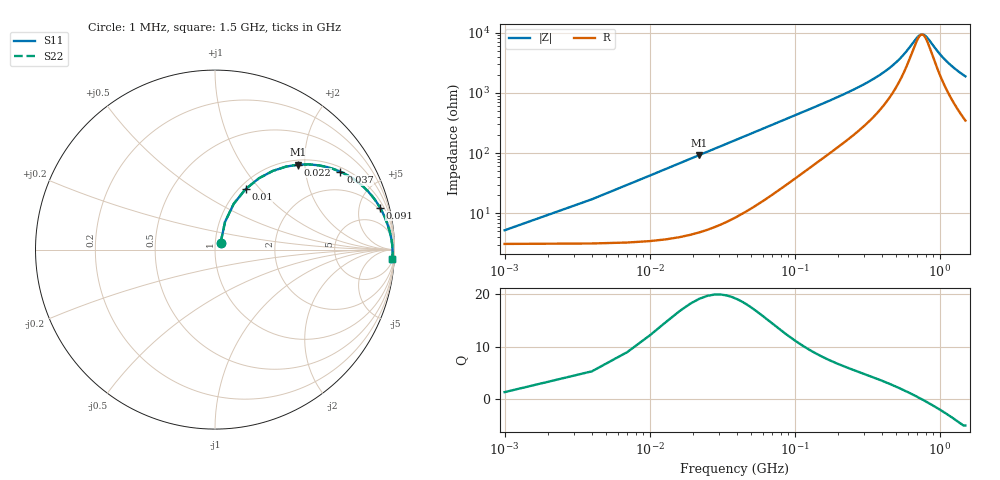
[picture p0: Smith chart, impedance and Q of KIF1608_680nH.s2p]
# MHz S RI R 50
!Freq ReS11 ImS11 ReS21 ImS21 ReS12 ImS12 ReS22 ImS22
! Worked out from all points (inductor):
!   501 points, 1 MHz to 1.5 GHz, reference 50 ohm
!   read as one part in series: L = 669 nH near 7 MHz
!   highest Q = 19.2 at 22 MHz (marker M1), where L = 669 nH
!   self-resonance near 750.9 MHz
!   S11 on the Smith chart (normalised r, x): 1 MHz: 1.06, +0.08; 10 MHz: 1.07, +0.84; 22 MHz: 1.10, +1.85; 37 MHz: 1.16, +3.11; 91 MHz: 1.64, +7.64; 1.5 GHz: 8, -37
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1  0.0317 0.0395  0.9683 -0.0395  0.9683 -0.0395  0.0317 0.0395
4  0.0557 0.154  0.9443 -0.154  0.9443 -0.154  0.0557 0.154
10  0.1704 0.3372  0.8296 -0.3372  0.8296 -0.3372  0.1704 0.3372
13  0.2453 0.3978  0.7547 -0.3978  0.7547 -0.3978  0.2453 0.3978
16  0.3221 0.4384  0.6779 -0.4384  0.6779 -0.4384  0.3221 0.4384
22  0.4637 0.4733  0.5363 -0.4733  0.5363 -0.4733  0.4637 0.4733
28  0.5776 0.4695  0.4224 -0.4695  0.4224 -0.4695  0.5776 0.4695
37  0.6988 0.4338  0.3012 -0.4338  0.3012 -0.4338  0.6988 0.4338
46  0.7771 0.3896  0.2229 -0.3896  0.2229 -0.3896  0.7771 0.3896
58  0.8416 0.3356  0.1584 -0.3356  0.1584 -0.3356  0.8416 0.3356
91  0.9193 0.2339  0.0807 -0.2339  0.0807 -0.2339  0.9193 0.2339
157  0.9613 0.1404  0.0387 -0.1404  0.0387 -0.1404  0.9613 0.1404
253  0.9773 0.0843  0.0227 -0.0843  0.0227 -0.0843  0.9773 0.0843
502  0.9874 0.0277  0.0126 -0.0277  0.0126 -0.0277  0.9874 0.0277
685  0.9891 0.00624  0.0109 -0.00624  0.0109 -0.00624  0.9891 0.00624
721  0.9893 0.00276  0.0107 -0.00276  0.0107 -0.00276  0.9893 0.00276
751  0.9894 -1.3e-05  0.0106 1.3e-05  0.0106 1.3e-05  0.9894 -1.3e-05
808  0.9895 -0.005  0.0105 0.005  0.0105 0.005  0.9895 -0.005
1003  0.9895 -0.0201  0.0105 0.0201  0.0105 0.0201  0.9895 -0.0201
1117  0.9892 -0.0279  0.0108 0.0279  0.0108 0.0279  0.9892 -0.0279
1252  0.9888 -0.0366  0.0112 0.0366  0.0112 0.0366  0.9888 -0.0366
1500  0.9876 -0.0513  0.0124 0.0513  0.0124 0.0513  0.9876 -0.0513
